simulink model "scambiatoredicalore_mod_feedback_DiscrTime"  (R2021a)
settings: Solver=FixedStepAuto  StartTime=0.0  StopTime=18000  FixedStep=Tsim  MaxStep=1  RelTol=1e-3
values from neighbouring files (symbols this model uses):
  ca = 4178    [scambiatoredicalore_dati.m]    (also in scambiatoremodelloTD.m)
  cb = 2131    [scambiatoredicalore_dati.m]    (also in scambiatoremodelloTD.m)
  ma = rhoa*pi*Di^2/4*L    (= 38.4179965995)    [scambiatoredicalore_dati.m]    (also in scambiatoremodelloTD.m)
  mb = rhob*pi*(Dan^2-De^2)/4*L    (= 72.0857488137)    [scambiatoredicalore_dati.m]    (also in scambiatoremodelloTD.m)
  Rba = Ri+Re+Rparete    [scambiatoredicalore_dati.m]    (also in scambiatoremodelloTD.m)
  Ta0 = 35    [scambiatoremodelloTD.m]
  Tain = 30    [scambiatoredicalore_dati.m]    (also in scambiatoremodelloTD.m)
  Tb0 = 55    [scambiatoremodelloTD.m]
  Tbin = 100    [scambiatoredicalore_dati.m]    (also in scambiatoremodelloTD.m)
  Tc = 10    [scambiatoremodelloTD.m]
  wa = 0.2    [scambiatoredicalore_dati.m]    (also in scambiatoremodelloTD.m)
  wb = 0.1    [scambiatoredicalore_dati.m]    (also in scambiatoremodelloTD.m)
undefined symbols (not defined in the file or in its folder): Kp, Tbin2, Tsim
libraries: pid_lib x1

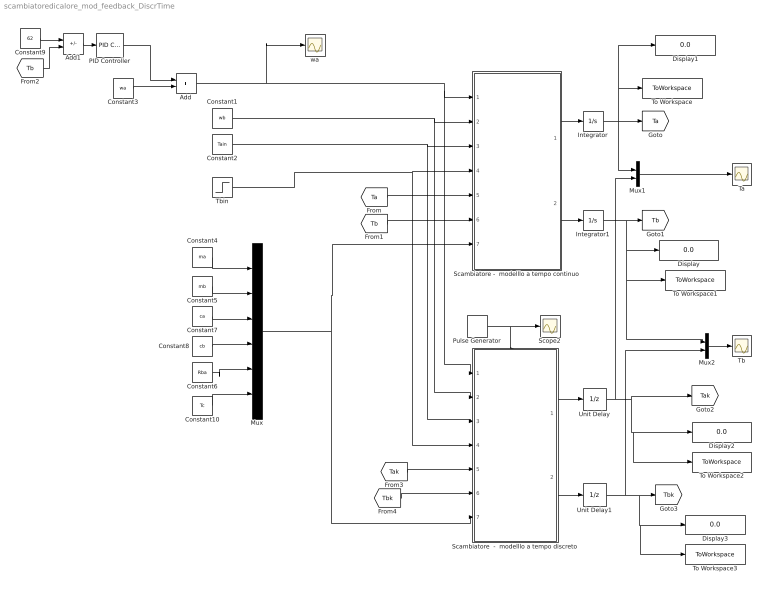
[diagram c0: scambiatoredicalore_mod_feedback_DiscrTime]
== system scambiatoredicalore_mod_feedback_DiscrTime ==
  Add : Sum
  Add1 : Sum  Inputs=-+
  Constant1 : Constant  Value=wb
  Constant10 : Constant  Value=Tc
  Constant2 : Constant  Value=Tain
  Constant3 : Constant  Value=wa
  Constant4 : Constant  Value=ma
  Constant5 : Constant  Value=mb
  Constant6 : Constant  Value=Rba
  Constant7 : Constant  Value=ca
  Constant8 : Constant  Value=cb
  Constant9 : Constant  Value=62
  Display{,1..3} (4 alike) : Display
  Integrator : Integrator  InitialCondition=Ta0
  Integrator1 : Integrator  InitialCondition=Tb0
  Mux : Mux  Inputs=6
  Mux1 : Mux  Inputs=2
  Mux2 : Mux  Inputs=2
  PID Controller : pid_lib/PID Controller  Controller=PID  Form=Parallel  TimeDomain=Continuous-time  UseExternalTs=off  SampleTime=-1  IntegratorMethod=Forward Euler  FilterMethod=Forward Euler  ControllerParametersSource=internal  P=Kp  I=0.0001  D=0  UseFilter=on  N=100  TunerSelectOption=Transfer Function Based (PID Tuner App)  InitialConditionSource=internal  InitialConditionForIntegrator=0  InitialConditionForFilter=0  DifferentiatorICPrevScaledInput=0  ExternalReset=none  TrackingMode=off  Kt=1  LimitOutput=off  SatLimitsSource=internal  UpperSaturationLimit=inf  LowerSaturationLimit=-inf  LinearizeAsGain=on  AntiWindupMode=none  Kb=1  POutMin=[]  POutMax=[]  IOutMin=[]  IOutMax=[]  DOutMin=[]  DOutMax=[]  NOutMin=[]  NOutMax=[]  SumOutMin=[]  SumOutMax=[]  SaturationOutMin=[]  SaturationOutMax=[]  PParamMin=[]  PParamMax=[]  IParamMin=[]  IParamMax=[]  DParamMin=[]  DParamMax=[]  NParamMin=[]  NParamMax=[]  KbParamMin=[]  KbParamMax=[]  KtParamMin=[]  KtParamMax=[]  KbOutMin=[]  KbOutMax=[]  KtOutMin=[]  KtOutMax=[]  IntegratorOutMin=[]  IntegratorOutMax=[]  FilterOutMin=[]  FilterOutMax=[]  SumI1OutMin=[]  SumI1OutMax=[]  SumI2OutMin=[]  SumI2OutMax=[]  SumI3OutMin=[]  SumI3OutMax=[]  SumI4OutMin=[]  SumI4OutMax=[]  SumDOutMin=[]  SumDOutMax=[]  DifferentiatorOutMin=[]  DifferentiatorOutMax=[]  FilterDiffOutCoefMin=[]  FilterDiffOutCoefMax=[]  ReciprocalOutMin=[]  ReciprocalOutMax=[]  SumDenOutMin=[]  SumDenOutMax=[]  SumNumOutMin=[]  SumNumOutMax=[]  DivideOutMin=[]  DivideOutMax=[]  UdiffTsProdOutMin=[]  UdiffTsProdOutMax=[]  NTsProdOutMin=[]  NTsProdOutMax=[]  UintegralTsProdOutMin=[]  UintegralTsProdOutMax=[]  UngainTsProdOutMin=[]  UngainTsProdOutMax=[]  IntegratorContinuousStateAttributes=''  IntegratorStateMustResolveToSignalObject=off  IntegratorRTWStateStorageClass=Auto  FilterContinuousStateAttributes=''  FilterStateMustResolveToSignalObject=off  FilterRTWStateStorageClass=Auto  ParallelPVariant=InternalParameters  IdealPVariant=Disabled  IVariant=InternalParameters  DVariant=InternalParameters  IntegratorVariant=Continuous  SatVariant=Disabled  AWVariant=Passthrough  PCopyVariant=Disabled  TRVariant=Disabled  FdbkBlocksVariant=Forward  IdealPFdbkVariant=Disabled  SatFdbkVariant=Disabled  DerivativeFilterVariant=ContFilter  NVariant=InternalParameters  NCopyVariant=Disabled  FilterICVariant=InternalICsFilter  IntegratorICVariant=InternalICs  ExternalResetVariant=Disabled  TRSumVariant=Passthrough  SumFdbkVariant=Disabled  SumVariant=Sum_PID  TsampFilterVariant=InternalTs  TsampNgainVariant=Passthrough  TsampIntegralVariant=Passthrough  ExternalSaturationOutDataTypeStr=Inherit: Same as second input
  Pulse Generator : DiscretePulseGenerator  PulseType=Time based  Period=Tc  PulseWidth=100*Tsim/Tc
  Scambiatore  -  modelllo a tempo discreto : Subsystem  TreatAsAtomicUnit=on
  Scambiatore -  modelllo a tempo continuo : MATLAB Function  TreatAsAtomicUnit=on
  Scope2 : Scope
  Ta : Scope
  Tb : Scope
  Tbin : Step  Time=10000  Before=Tbin  After=Tbin2  SampleTime=0
  To Workspace : ToWorkspace  VariableName=TaTC  SaveFormat=Timeseries  SampleTime=-1
  To Workspace1 : ToWorkspace  VariableName=TbTC  SaveFormat=Timeseries  SampleTime=-1
  To Workspace2 : ToWorkspace  VariableName=Tak  SaveFormat=Timeseries  SampleTime=-1
  To Workspace3 : ToWorkspace  VariableName=Tbk  SaveFormat=Timeseries  SampleTime=-1
  Unit Delay : UnitDelay  InitialCondition=Ta0  SampleTime=Tc  HasFrameUpgradeWarning=on
  Unit Delay1 : UnitDelay  InitialCondition=Tb0  SampleTime=Tc  HasFrameUpgradeWarning=on
  wa : Scope
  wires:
  Scambiatore -  modelllo a tempo continuo/1(Tadot) -> Integrator/1
  Scambiatore -  modelllo a tempo continuo/2(Tbdot) -> Integrator1/1
  Integrator/1 -> [Ta], Display1/1, To Workspace/1, Mux1/1
  Integrator1/1 -> Display/1, Mux2/1, To Workspace1/1, [Tb]
  [Tb] -> Scambiatore -  modelllo a tempo continuo/6(Tb)
  Add/1 -> wa/1, Scambiatore  -  modelllo a tempo discreto/1(wa), Scambiatore -  modelllo a tempo continuo/1(wa)
  Constant1/1 -> Scambiatore  -  modelllo a tempo discreto/2(wb), Scambiatore -  modelllo a tempo continuo/2(wb)
  Constant2/1 -> Scambiatore  -  modelllo a tempo discreto/3(Tain), Scambiatore -  modelllo a tempo continuo/3(Tain)
  Tbin/1 -> Scambiatore -  modelllo a tempo continuo/4(Tbin), Scambiatore  -  modelllo a tempo discreto/4(Tbin)
  Constant4/1 -> Mux/1
  Constant5/1 -> Mux/2
  Mux/1 -> Scambiatore -  modelllo a tempo continuo/7(par), Scambiatore  -  modelllo a tempo discreto/7(par)
  Constant7/1 -> Mux/3
  Constant8/1 -> Mux/4
  Constant6/1 -> Mux/5
  Mux1/1 -> Ta/1
  Constant3/1 -> Add/2
  [Tb] -> Add1/2
  Constant9/1 -> Add1/1
  Add1/1 -> PID Controller/1
  PID Controller/1 -> Add/1
  Unit Delay/1 -> Mux1/2, To Workspace2/1, Display2/1, [Tak]
  [Ta] -> Scambiatore -  modelllo a tempo continuo/5(Ta)
  Unit Delay1/1 -> Mux2/2, To Workspace3/1, Display3/1, [Tbk]
  Constant10/1 -> Mux/6
  [Tak] -> Scambiatore  -  modelllo a tempo discreto/5(Tak)
  [Tbk] -> Scambiatore  -  modelllo a tempo discreto/6(Tbk)
  Scambiatore  -  modelllo a tempo discreto/1(Takp1) -> Unit Delay/1
  Scambiatore  -  modelllo a tempo discreto/2(Tbkp1) -> Unit Delay1/1
  Pulse Generator/1 -> Scope2/1, Scambiatore  -  modelllo a tempo discreto/Enable
  Mux2/1 -> Tb/1

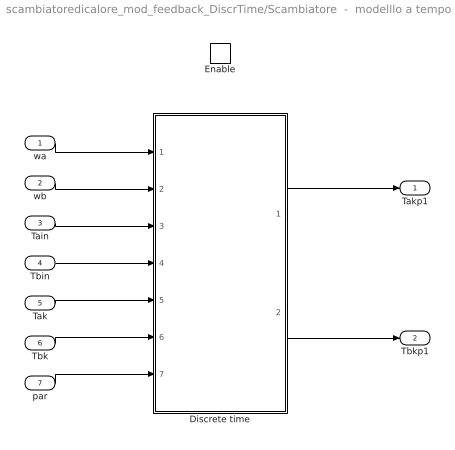
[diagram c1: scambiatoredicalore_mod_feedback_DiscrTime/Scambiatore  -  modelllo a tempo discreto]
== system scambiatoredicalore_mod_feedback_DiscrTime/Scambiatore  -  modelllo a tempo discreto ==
  wa : Inport
  wb : Inport  Port=2
  Tain : Inport  Port=3
  Tbin : Inport  Port=4
  Tak : Inport  Port=5
  Tbk : Inport  Port=6
  par : Inport  Port=7
  Enable : EnablePort
  Discrete time : MATLAB Function  TreatAsAtomicUnit=on
  Takp1 : Outport
  Tbkp1 : Outport  Port=2
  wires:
  par/1 -> Discrete time/7(par)
  Discrete time/1(Takp1) -> Takp1/1
  Tbk/1 -> Discrete time/6(Tbk)
  Discrete time/2(Tbkp1) -> Tbkp1/1
  wb/1 -> Discrete time/2(wb)
  Tain/1 -> Discrete time/3(Tain)
  Tbin/1 -> Discrete time/4(Tbin)
  wa/1 -> Discrete time/1(wa)
  Tak/1 -> Discrete time/5(Tak)

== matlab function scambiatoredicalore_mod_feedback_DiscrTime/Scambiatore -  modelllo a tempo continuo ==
function [Tadot,Tbdot] = fcn(wa,wb,Tain,Tbin,Ta,Tb,par)

ma=par(1);
mb=par(2);
ca=par(3);
cb=par(4);
Rba=par(5);

DT1=Tbin-Ta;
DT2=Tb-Tain;

Tadot =  1/ma*wa*(Tain-Ta)+1/(Rba*ma*ca)*(DT1-DT2)/log(DT1/DT2);
Tbdot =  1/mb*wb*(Tbin-Tb)-1/(Rba*mb*cb)*(DT1-DT2)/log(DT1/DT2);

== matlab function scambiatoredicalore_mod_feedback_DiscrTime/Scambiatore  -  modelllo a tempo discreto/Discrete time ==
function [Takp1,Tbkp1] = fcn(wa,wb,Tain,Tbin,Tak,Tbk,par)

ma=par(1);
mb=par(2);
ca=par(3);
cb=par(4);
Rba=par(5);
Tc=par(6);

DT1=Tbin-Tak;
DT2=Tbk-Tain;

Takp1 = Tak+Tc*( 1/ma*wa*(Tain-Tak)+1/(Rba*ma*ca)*(DT1-DT2)/log(DT1/DT2) );
Tbkp1 = Tbk+Tc*( 1/mb*wb*(Tbin-Tbk)-1/(Rba*mb*cb)*(DT1-DT2)/log(DT1/DT2) );
